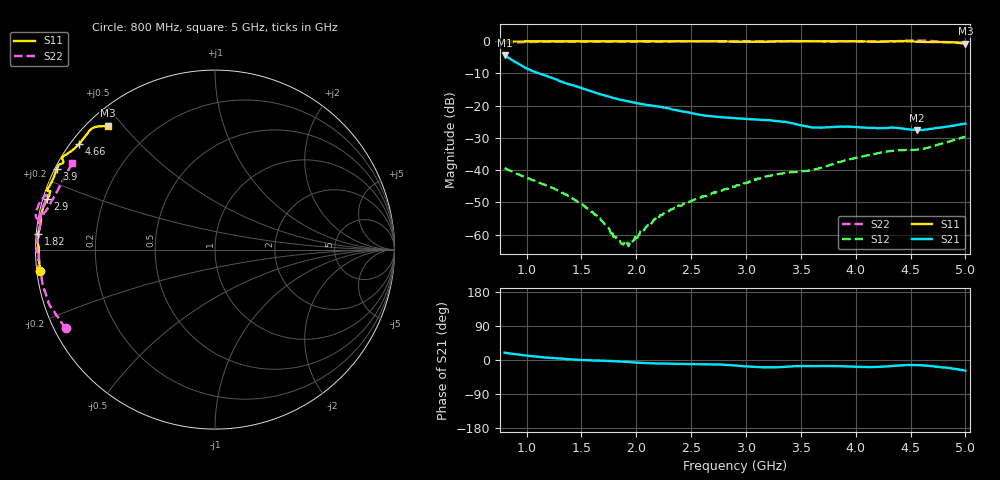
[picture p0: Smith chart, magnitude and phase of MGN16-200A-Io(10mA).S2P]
! Port[1] = GATE
! Port[2] = DRAIN
! [Type]  S-parameter s2p file
! [Object]  MGN16-200A
! [Bias]  10 mA
! [Version]  1.0
! [Date]  Jul 2026
! [Source]  This file was created in JSC "ICC Milandr".
! [Disclaimer] Property of JSC "ICC Milandr". Unauthorized reproduction and/or distribution is strictly prohibited.
!  The file and the data are provided "AS IS" and with all faults and disclaim all warranties, express and implied, including
!  without limitation any implied warranties of merchantability, fitness for a particular purpose.
!  JSC "ICC Milandr" assumes no liability for:
!  1) the accuracy of the data provided;
!  2) the proper functioning of this data;
!  3) infringement of patents, copyrights or intellectual property rights resulting from the use of this data.
!  JSC "ICC Milandr" reserves the right to make changes to the products and the data without prior notice.
!  Please, be aware that your receipt and use of the file provided shall serve as acceptance of these terms and conditions.
!  If you do not accept these terms, you should return or destroy this file and any other accompanying information immediately.
# GHZ S MA R 50
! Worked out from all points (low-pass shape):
!   421 points, 800 MHz to 5 GHz, reference 50 ohm
!   highest |S21| = -4.32 dB at 800 MHz (marker M1); lowest = -27.6 dB at 4.56 GHz (marker M2)
!   |S21| within 3 dB of the highest: start of sweep to 938 MHz
!   lowest |S11| = -0.8 dB at 5 GHz (marker M3), VSWR 21.88, Z = 2.76 + j22.8 ohm
!   |S11| at or under -10 dB: nowhere
!   |S22| runs from -0.6 to 0.2 dB; largest |S21 - S12| = 0.61
!   S11 on the Smith chart (normalised r, x): 800 MHz: 0.01, -0.06; 1.82 GHz: 0.01, +0.04; 2.9 GHz: 0.01, +0.15; 3.9 GHz: 0.01, +0.24; 4.66 GHz: 0.02, +0.34; 5 GHz: 0.06, +0.46
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0.8  0.9793 -173.1  0.6079 19.3  0.01074 -64.5  0.9397 -152.1
1.05  0.9817 -178.6  0.3445 10.0  0.006951 -71.2  0.9658 -160.0
1.26  0.984 178.7  0.2576 4.8  0.005058 -74.8  0.9731 -163.9
1.5  0.9888 177.8  0.1867 -0.0  0.003022 -72.2  0.9794 -169.0
1.68  0.9888 176.7  0.1485 -1.6  0.001674 -65.6  0.979 -171.9
1.82  0.9886 175.0  0.1277 -3.3  0.0009029 -42.2  0.9786 -173.1
1.89  0.9868 173.7  0.1197 -4.5  0.0007425 -13.7  0.9827 -173.6
1.95  0.9847 172.7  0.114 -5.6  0.0007639 16.8  0.9877 -174.0
2.06  0.9829 171.0  0.1046 -7.8  0.00122 46.6  0.9927 -174.9
2.2  0.9849 170.1  0.09634 -9.1  0.001771 55.0  0.9845 -177.0
2.45  0.9902 169.7  0.07984 -10.6  0.00309 65.5  0.9891 179.9
2.9  0.9755 163.3  0.06361 -14.4  0.005502 72.0  0.994 179.2
3.17  0.9763 160.6  0.0595 -19.4  0.00779 67.0  0.9859 174.4
3.38  0.9911 160.7  0.05496 -17.6  0.009135 69.4  0.9841 169.9
3.6  0.9881 159.1  0.04587 -16.2  0.009976 70.3  0.994 171.0
3.9  0.9904 153.0  0.04692 -16.5  0.01412 68.3  0.9916 170.4
4.3  0.9847 149.6  0.04491 -16.6  0.01947 58.3  0.9813 162.1
4.42  0.9948 148.8  0.04408 -13.8  0.02041 58.8  1.001 163.4
4.56  0.9768 146.4  0.04156 -13.7  0.02065 56.2  1.017 168.2
4.66  0.9594 142.3  0.04277 -15.3  0.02213 53.2  1.007 170.1
4.8  0.9633 136.3  0.04622 -19.9  0.02624 46.6  0.9615 166.4
5  0.9126 130.9  0.05253 -28.2  0.03281 34.0  0.9285 148.8
